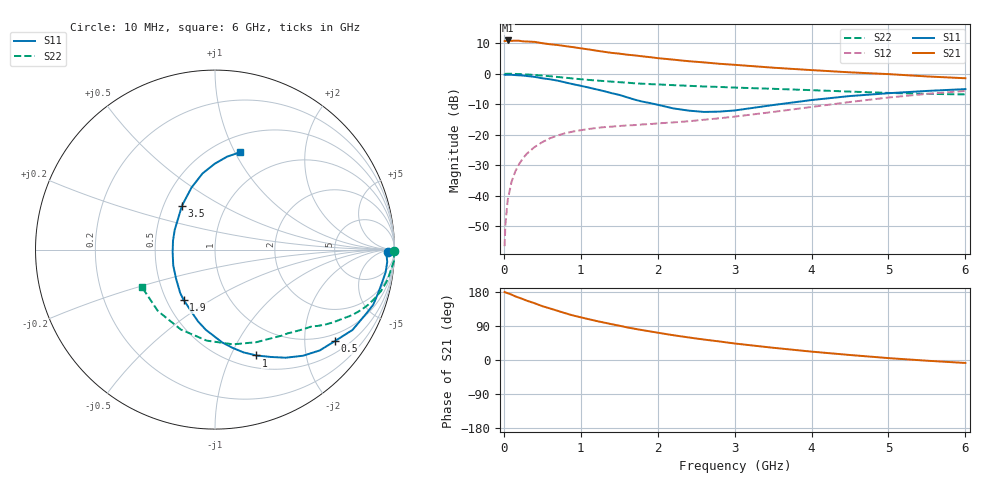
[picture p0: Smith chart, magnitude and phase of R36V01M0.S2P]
! SIEMENS Small Signal Semiconductors
! BFR181
! Si NPN RF Bipolar Junction Transistor in SOT23
! VCE = 6 V  IC = 1 mA
! Common Emitter S-Parameters:  May  1996
# GHz  S  MA  R  50
!  f  S11  S21  S12  S22
! GHz  MAG  ANG  MAG  ANG  MAG  ANG  MAG  ANG
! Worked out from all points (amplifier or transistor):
!   36 points, 10 MHz to 6 GHz, reference 50 ohm
!   highest |S21| = 10.9 dB at 50 MHz (marker M1)
!   |S21| within 3 dB of that: start of sweep to 1.117 GHz
!   unconditionally stable (mu >= 1): 2.053 GHz to 3.675 GHz
!   at 250 MHz: K = 0.15, MSG = 19.1 dB, |S12| = -27.7 dB
!   at 1.4 GHz: K = 0.76, MSG = 12.1 dB, |S12| = -17.3 dB
!   at 6 GHz: K = 0.87, MSG = 2.1 dB, |S12| = -5.6 dB
!   lowest NFmin = 1.30 dB at 450 MHz
!   S11 on the Smith chart (normalised r, x): 10 MHz: 44, -18; 500 MHz: 0.80, -2.77; 1 GHz: 0.64, -1.26; 1.9 GHz: 0.61, -0.38; 3.5 GHz: 0.62, +0.34; 6 GHz: 0.66, +1.05
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0.01  0.9617 -0.9  3.432 179.3  0.0015 92.4  0.9985 -0.4
0.02  0.9554 -1.4  3.416 178.3  0.0033 92.4  0.9923 -0.7
0.05  0.962 -4.1  3.5 176.3  0.0085 87.7  0.9972 -1.8
0.1  0.9589 -7.6  3.454 172.6  0.017 85.2  0.9988 -3.6
0.15  0.948 -11.5  3.474 167.8  0.0253 82.1  0.9907 -5.5
0.2  0.9399 -15.4  3.461 164.3  0.0333 80.0  0.9845 -7.2
0.4  0.8873 -30.3  3.316 149.8  0.0631 70.5  0.9535 -14.0
0.5  0.8411 -37.2  3.155 142.1  0.0757 66.5  0.9302 -17.0
0.7  0.7685 -50.3  2.946 129.7  0.0974 59.4  0.8837 -22.2
0.8  0.7191 -56.9  2.828 123.4  0.1061 56.3  0.8591 -24.4
1  0.6334 -68.6  2.6 112.6  0.1187 51.3  0.8111 -28.2
1.1  0.5944 -74.5  2.497 107.9  0.1243 49.6  0.7913 -29.9
1.4  0.4804 -90.9  2.192 94.5  0.1359 45.6  0.7413 -34.4
1.7  0.376 -109.6  1.994 82.4  0.144 44.7  0.6961 -37.8
1.9  0.3305 -121.9  1.865 75.5  0.1496 44.8  0.6749 -40.2
2.2  0.2706 -143.3  1.7 65.5  0.1592 45.7  0.6494 -43.9
2.6  0.2364 -176.6  1.531 54.0  0.176 48.2  0.6175 -49.1
3  0.25 153.9  1.398 43.6  0.1982 50.4  0.5924 -55.5
3.5  0.3067 126.8  1.254 32.3  0.2363 51.6  0.5653 -65.8
4.5  0.4306 99.2  1.052 13.2  0.3442 47.5  0.5092 -95.2
5.5  0.5221 82.6  0.902 -1.9  0.4669 35.4  0.4673 -132.9
6  0.5594 75.7  0.842 -7.8  0.5221 27.5  0.4578 -153.1
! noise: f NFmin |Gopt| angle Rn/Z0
0.45  1.3  0.7  18  0.5
0.9  1.4  0.6  39  0.52
1.8  1.85  0.4  81  0.47
